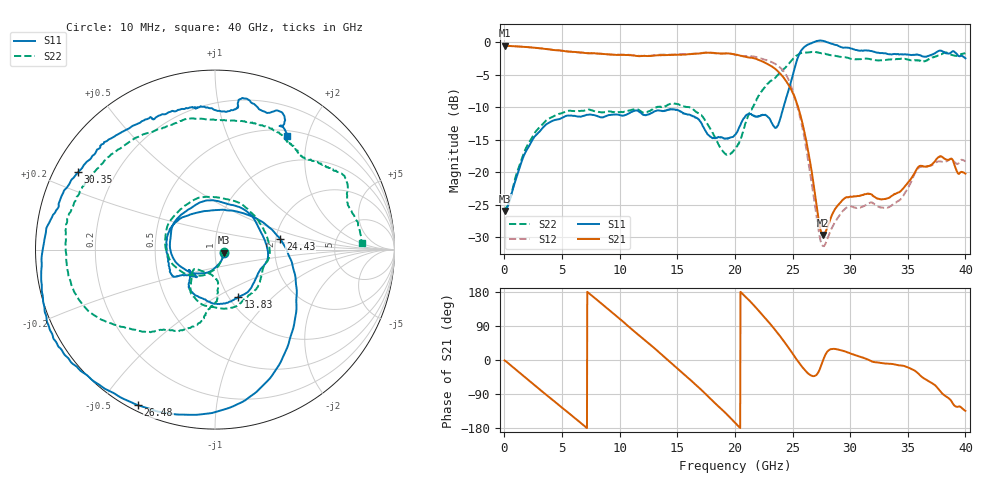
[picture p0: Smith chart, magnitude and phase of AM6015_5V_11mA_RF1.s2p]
!Agilent Technologies,E8364B,MY43040894,A.07.50.67
!Agilent E8364B: A.07.50.67
!Date: Wednesday, May 01, 2019 08:18:05
!Correction: S11(Full 2 Port(1,2))
!S21(Full 2 Port(1,2))
!S12(Full 2 Port(1,2))
!S22(Full 2 Port(1,2))
!S2P File: Measurements: S11, S21, S12, S22:
# Hz S  dB  R 50
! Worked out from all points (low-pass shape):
!   1601 points, 10 MHz to 40 GHz, reference 50 ohm
!   highest |S21| = -0.58 dB at 10 MHz (marker M1); lowest = -29.6 dB at 27.63 GHz (marker M2)
!   |S21| within 3 dB of the highest: start of sweep to 23.03 GHz
!   lowest |S11| = -26.0 dB at 10 MHz (marker M3), VSWR 1.11, Z = 55 - j1.84 ohm
!   |S11| at or under -10 dB: start of sweep to 24.22 GHz
!   |S22| runs from -25.6 to -1.5 dB; largest |S21 - S12| = 0.093
!   S11 on the Smith chart (normalised r, x): 10 MHz: 1.10, -0.04; 13.83 GHz: 1.10, -0.64; 24.43 GHz: 2.12, +0.29; 26.48 GHz: 0.02, -0.62; 30.35 GHz: 0.07, +0.26; 40 GHz: 0.58, +1.67
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1e7  -25.96 -19.4  -0.58 -1.2  -0.48 -2.2  -25.63 -14.7
3.309175e9  -13.20 -156.4  -1.02 -84.1  -1.01 -84.0  -12.61 -153.1
4.8088e9  -11.80 164.1  -1.28 -121.1  -1.31 -121.1  -10.99 170.6
6.683331e9  -11.43 118.6  -1.63 -167.7  -1.62 -167.6  -10.55 124.7
8.282931e9  -11.52 79.7  -1.82 152.1  -1.80 152.3  -10.75 82.9
1.028243e10  -11.30 25.4  -1.98 101.4  -1.95 101.5  -10.75 29.3
1.335666e10  -10.51 -53.7  -2.04 22.0  -1.97 21.9  -9.97 -44.7
1.383154e10  -10.60 -64.0  -2.02 9.2  -1.92 9.0  -9.93 -55.8
1.540615e10  -10.78 -99.2  -1.93 -32.9  -1.89 -33.4  -9.79 -88.5
1.730568e10  -13.20 -130.1  -1.69 -85.3  -1.63 -85.3  -11.75 -121.9
2.0005e10  -14.25 -130.1  -1.91 -165.5  -1.96 -165.3  -16.37 -93.1
2.132967e10  -11.07 -152.6  -2.41 154.4  -2.17 155.6  -10.75 -88.8
2.260435e10  -11.18 156.6  -3.17 111.2  -2.72 111.9  -6.91 -107.0
2.442889e10  -8.66 9.2  -5.97 41.9  -5.01 34.6  -3.84 -136.4
2.532867e10  -3.09 -56.7  -9.16 2.7  -9.31 -9.1  -2.10 -154.2
2.647838e10  -0.28 -116.3  -17.94 -38.7  -19.58 -48.2  -1.60 176.6
2.667833e10  -0.16 -126.3  -20.08 -41.7  -21.86 -49.4  -1.52 172.6
2.762809e10  0.17 -155.0  -29.61 -2.2  -31.31 -4.3  -1.77 155.3
3.035241e10  -1.14 150.6  -23.68 13.6  -25.39 17.6  -2.64 113.0
3.335166e10  -1.89 115.4  -23.94 -10.1  -25.38 2.7  -2.67 77.1
3.777556e10  -1.33 79.5  -17.54 -80.6  -18.32 -60.9  -2.01 34.1
4e10  -2.51 57.4  -20.22 -134.0  -18.36 -116.6  -1.72 2.7
